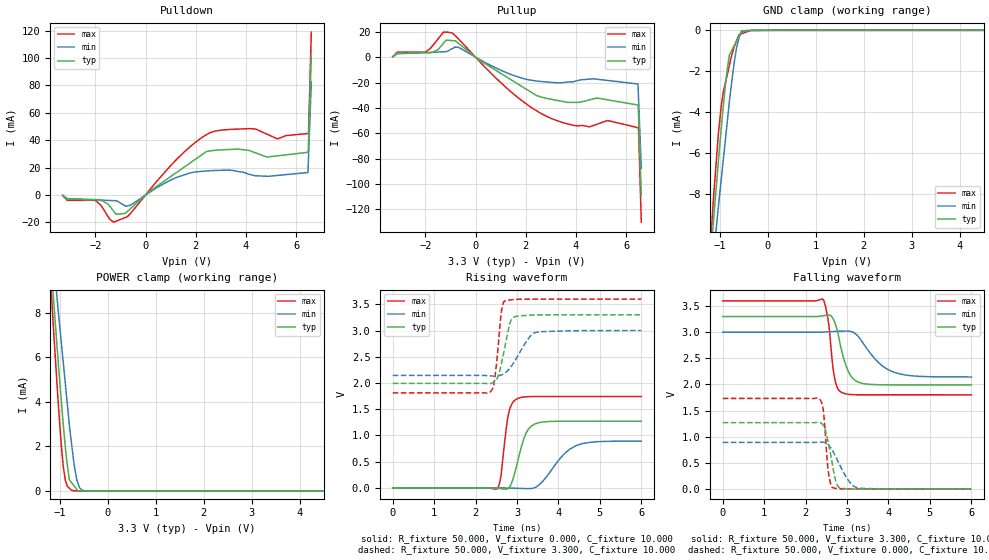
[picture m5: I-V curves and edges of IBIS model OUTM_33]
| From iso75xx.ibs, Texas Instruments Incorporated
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|   OUTM_33 MODEL
[Model]   OUTM_33
Model_type   3-state
Polarity   Non-Inverting
Vmeas = 1.65
Vref = 1.65
Cref = 15pF
Rref = 50
|   typ   min   max
| High state   (typ PVT)   (Fast PVT)   (Slow PVT)
C_comp   1.5262p   1.2349p   1.8603p
|C_comp (Low state)   1.5194p   1.2295p   1.8511p
[Voltage Range]   3.3   3   3.6
[Temperature Range]   27   125   -40
[Pullup Reference]   3.3   3   3.6
[Pulldown Reference]   -0   -0   -0
[Power Clamp Reference]   3.3   3   3.6
[GND Clamp Reference]   -0   -0   -0
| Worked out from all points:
|   slope of the pulldown table from 0 to 0.495 V, typ, clamps not added: 72.6 ohm
|   slope of the pullup table from 0 to 0.495 V, typ, clamps not added: 76 ohm
|   GND clamp passes 1 mA (typ) near -0.76 V on its own axis
|   POWER clamp passes 1 mA (typ) near -0.83 V on its own axis
|   falling waveform, R_fixture 50.000, V_fixture 3.300, C_fixture 10.000: 20-80 % time 265ps typ, 571ps min, 150ps max; typ from 3.3 V to 1.99 V
|   rising waveform, R_fixture 50.000, V_fixture 0.000, C_fixture 10.000: 20-80 % time 272ps typ, 558ps min, 161ps max; typ from -0.003 V to 1.27 V
|   rising waveform, R_fixture 50.000, V_fixture 3.300, C_fixture 10.000: 20-80 % time 209ps typ, 400ps min, 128ps max; typ from 1.99 V to 3.3 V
|   falling waveform, R_fixture 50.000, V_fixture 0.000, C_fixture 10.000: 20-80 % time 184ps typ, 358ps min, 104ps max; typ from 1.27 V to -0.003 V
[Pulldown]
|   Voltage   I(typ)   I(min)   I(max)
-3.3V     -334.5uA   -211.2uA   -377.3uA
-3.126V   -3.089mA   -2.632mA   -3.962mA
-2.017V   -3.408mA   -3.584mA   -3.917mA
-1.278V   -11.74mA   -4.178mA   -19.91mA
-645.9mV  -10.8mA    -7.75mA    -14.4mA
1.151V    15.36mA    12.08mA    24.34mA
2.528V    32.04mA    17.65mA    45.07mA
4.215V    31.87mA    14.68mA    48.4mA
5.253V    28.55mA    14.23mA    40.94mA
6.466V    31.13mA    16.35mA    44.85mA
6.488V    37.87mA    26.93mA    44.89mA
6.6V      101.8mA    82.49mA    118.9mA
[GND Clamp]
|   Voltage   I(typ)   I(min)   I(max)
-3.3V     -68.19mA   -59mA      -79.06mA
-1.174V   -10.48mA   -12.05mA   -9.647mA
-1.124V   -9.051mA   -10.85mA   -7.908mA
-1.037V   -6.541mA   -8.744mA   -5.226mA
-971.1mV  -4.786mA   -7.274mA   -3.677mA
-869.3mV  -2.326mA   -4.994mA   -2.404mA
-804.1mV  -1.221mA   -3.532mA   -1.732mA
-701.2mV  -740.2uA   -1.566mA   -800uA
-645.9mV  -481.7uA   -774.6uA   -474.7uA
-547.9mV  -23.95uA   -123.4uA   -165.3uA
-349.9mV  -16.77uA   -877nA     -90.86nA
6.6V      0A         0A         0A
[Pullup]
|   Voltage   I(typ)   I(min)   I(max)
-3.3V     324uA      217.7uA    399uA
-2.017V   3.409mA    3.671mA    3.907mA
-1.278V   11.06mA    4.308mA    19.85mA
-929.5mV  13.13mA    6.764mA    19.15mA
-645.9mV  10.4mA     7.454mA    13.68mA
1.286V    -16.24mA   -12.65mA   -25.17mA
2.865V    -32.65mA   -19.62mA   -47.04mA
4.055V    -35.68mA   -18.47mA   -54.26mA
5.253V    -33.64mA   -18.34mA   -49.99mA
6.466V    -37.78mA   -21.14mA   -55.6mA
6.488V    -44.59mA   -31.8mA    -55.7mA
6.6V      -108.9mA   -87.75mA   -130.3mA
[POWER Clamp]
|   Voltage   I(typ)   I(min)   I(max)
-3.3V     67.74mA    58.5mA     78.64mA
-1.174V   9.821mA    11.44mA    8.772mA
-1.124V   8.384mA    10.24mA    6.981mA
-1.037V   5.859mA    8.143mA    4.035mA
-929.5mV  2.988mA    5.776mA    1.104mA
-887.9mV  2.019mA    4.857mA    496.1uA
-804.1mV  504.3uA    3.008mA    124uA
-763.1mV  390.6uA    2.237mA    34.85uA
-645.9mV  65.69uA    486.1uA    3.089uA
-590.6mV  2.481uA    143.9uA    266.5nA
-479.9mV  2.091uA    7.048uA    144nA
6.6V      0A         0A         0A
[Ramp]
R_load = 50
|   typ   min   max
dV/dt_r   0.796291/2.70925e-10   0.534731/5.58911e-10   1.045/1.61806e-10
dV/dt_f   0.840769/2.65072e-10   0.514276/5.72621e-10   1.07919/1.50749e-10
[Falling Waveform]
R_fixture = 50.000
V_fixture = 3.300
V_fixture_min = 3.000
V_fixture_max = 3.600
C_fixture = 10.000
|  time   V(typ)   V(min)   V(max)
0s        3.3V       3V         3.6V
2.411ns   3.313V     3.002V     3.634V
2.542ns   3.327V     3.008V     3.241V
2.703ns   3.189V     3.015V     2.117V
2.886ns   2.596V     3.021V     1.841V
3.068ns   2.193V     3.019V     1.809V
3.354ns   2.024V     2.83V      1.803V
3.766ns   1.995V     2.414V     1.802V
4.151ns   1.992V     2.229V     1.802V
6ns       1.992V     2.143V     1.801V
[Rising Waveform]
R_fixture = 50.000
V_fixture = 0.000
V_fixture_min = 0.000
V_fixture_max = 0.000
C_fixture = 10.000
|  time   V(typ)   V(min)   V(max)
0s        -3.409mV   2.641nV    1.959nV
2.52ns    -11.36mV   -389.9uV   -15.81mV
2.606ns   -15.9mV    -1.26mV    192.9mV
2.735ns   -25.1mV    -3.344mV   1.099V
2.805ns   -679.6uV   -4.797mV   1.445V
3.035ns   563.2mV    -9.583mV   1.71V
3.221ns   1.048V     -14.84mV   1.736V
3.505ns   1.238V     40.68mV    1.742V
4.439ns   1.27V      808.7mV    1.742V
6ns       1.27V      891.2mV    1.742V
[Rising Waveform]
R_fixture = 50.000
V_fixture = 3.300
V_fixture_min = 3.000
V_fixture_max = 3.600
C_fixture = 10.000
|  time   V(typ)   V(min)   V(max)
0s        1.992V     2.143V     1.811V
2.35ns    1.988V     2.135V     1.828V
2.454ns   2.02V      2.132V     2.035V
2.617ns   2.343V     2.151V     3.316V
2.707ns   2.688V     2.187V     3.563V
2.83ns    3.142V     2.284V     3.582V
2.886ns   3.235V     2.346V     3.587V
3.244ns   3.289V     2.814V     3.599V
3.461ns   3.296V     2.966V     3.599V
6ns       3.3V       3V         3.6V
[Falling Waveform]
R_fixture = 50.000
V_fixture = 0.000
V_fixture_min = 0.000
V_fixture_max = 0.000
C_fixture = 10.000
|  time   V(typ)   V(min)   V(max)
0s        1.27V      890.3mV    1.733V
2.332ns   1.273V     896.6mV    1.724V
2.426ns   1.218V     894.7mV    1.519V
2.538ns   925.1mV    852.6mV    402.1mV
2.594ns   704.4mV    803.7mV    129.6mV
2.657ns   427.9mV    724.2mV    24.07mV
2.8ns     34.83mV    498.8mV    6.443mV
3.052ns   2.327mV    143.9mV    549.9uV
3.244ns   -1.415mV   23.34mV    123.4uV
6ns       -3.409mV   1.688uV    5.148nV
